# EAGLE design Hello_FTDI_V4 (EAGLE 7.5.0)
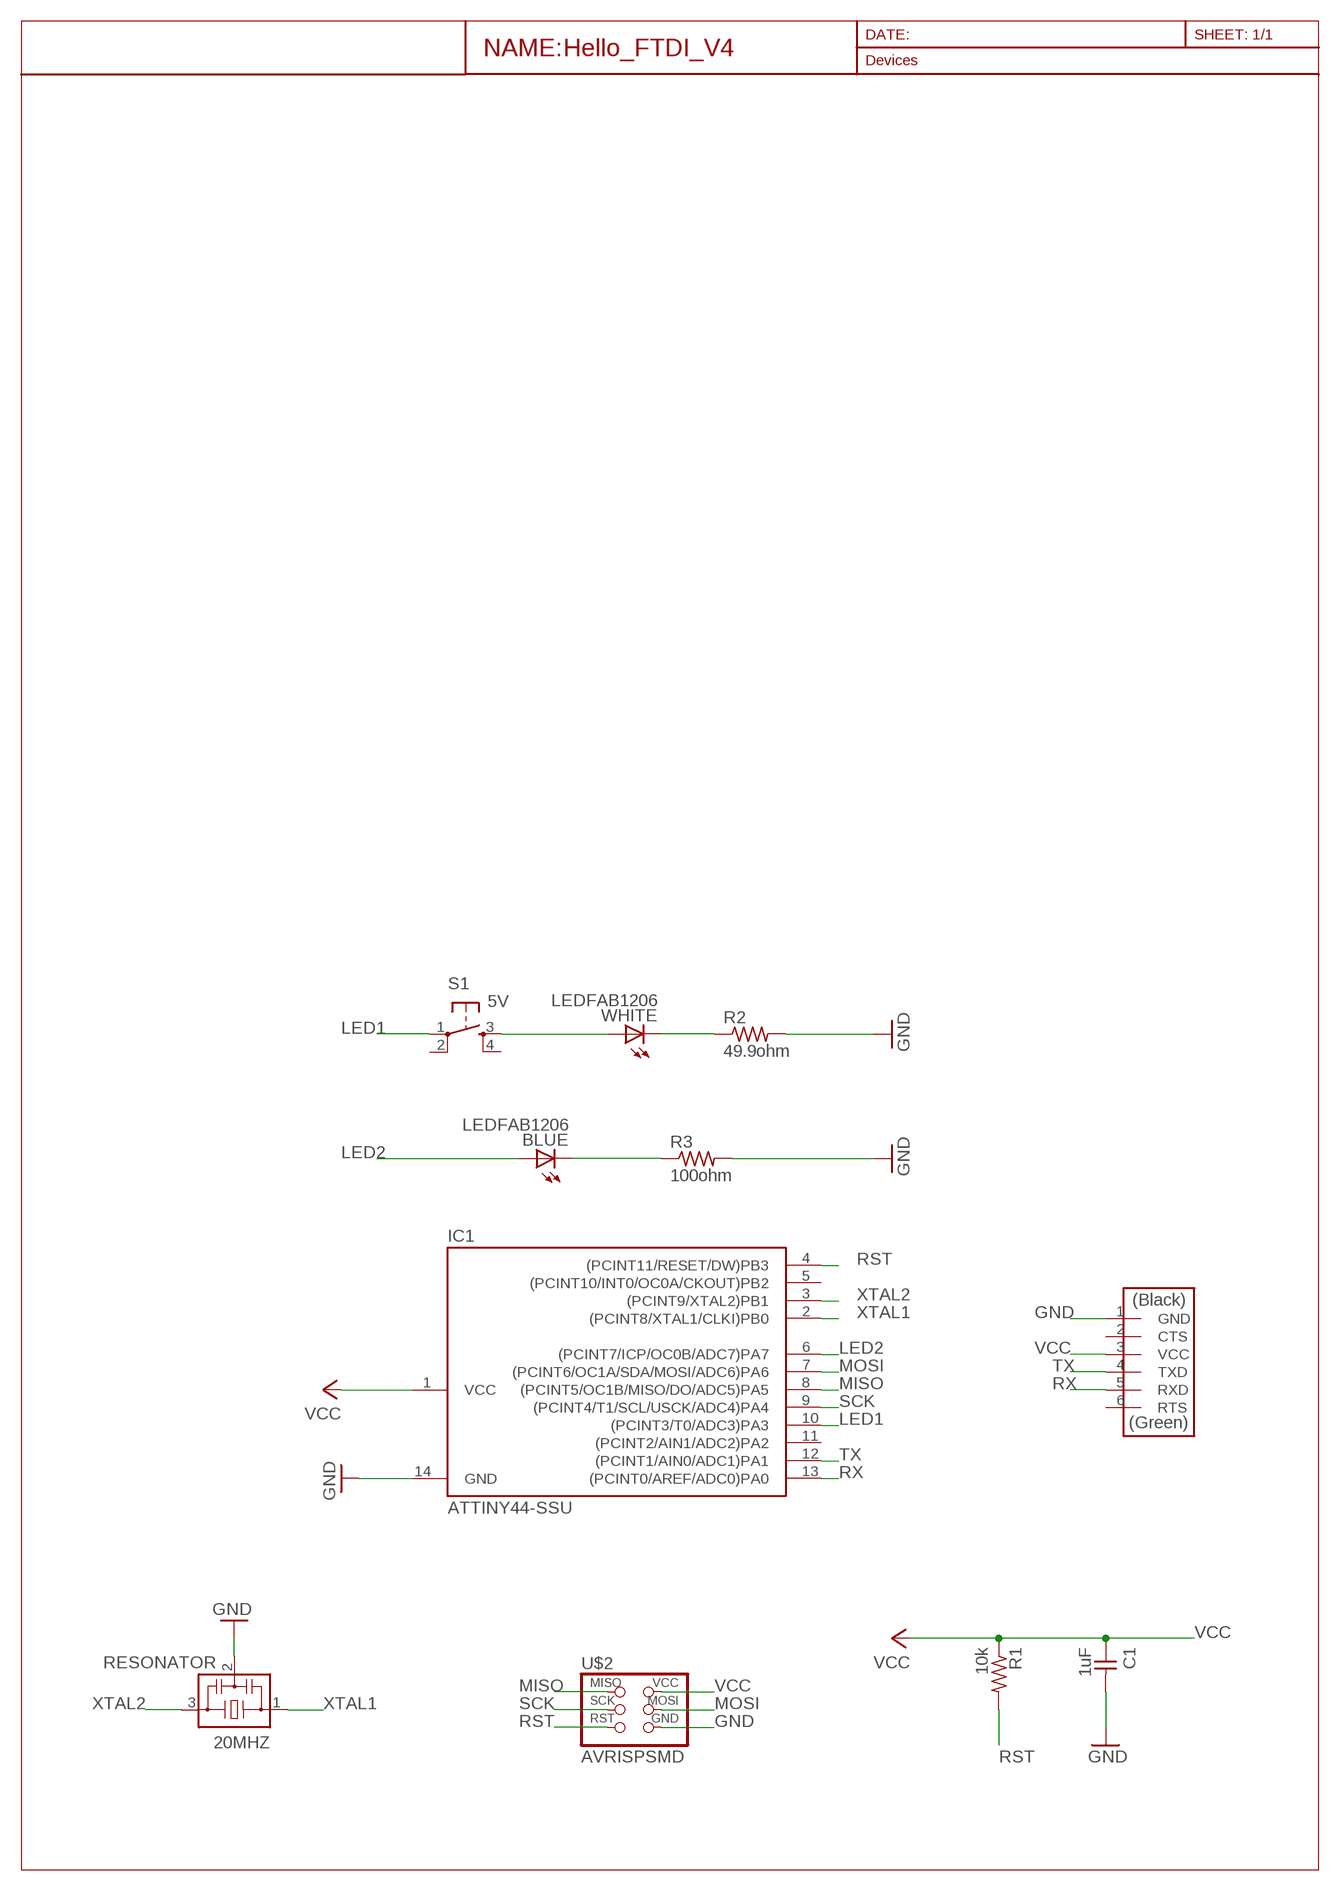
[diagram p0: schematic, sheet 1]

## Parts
20MHZ  RESONATOR  [EFOBM]
BLUE  LEDFAB1206  [LED1206FAB]
C1  1uF  CAP-UNPOLARIZEDFAB  [C1206FAB]
FTDI  FTDI-SMD-HEADER  [1X06SMD]
IC1  ATTINY44-SSU  [SOIC14]
R1  10k  RES-US1206FAB  [R1206FAB]
R2  49.9ohm  RES-US1206FAB  [R1206FAB]
R3  100ohm  RES-US1206FAB  [R1206FAB]
S1  5V  6MM_SWITCH6MM_SWITCH  [6MM_SWITCH]
U$2  AVRISPSMD  [2X03SMD]
WHITE  LEDFAB1206  [LED1206FAB]

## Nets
GND: 20MHZ.2 C1.2 FTDI.1(GND) IC1.14(GND) R2.2 R3.2 U$2.6(GND)
LED1: IC1.10((PCINT3/T0/ADC3)PA3) S1.1(P)
LED2: BLUE.1(A) IC1.6((PCINT7/ICP/OC0B/ADC7)PA7)
MISO: IC1.8((PCINT5/OC1B/MISO/DO/ADC5)PA5) U$2.1(MISO)
MOSI: IC1.7((PCINT6/OC1A/SDA/MOSI/ADC6)PA6) U$2.4(MOSI)
N$1: R2.1 WHITE.2(C)
N$2: S1.3(S) WHITE.1(A)
N$3: BLUE.2(C) R3.1
RST: IC1.4((PCINT11/RESET/DW)PB3) R1.2 U$2.5(RST)
RX: FTDI.5(RXD) IC1.13((PCINT0/AREF/ADC0)PA0)
SCK: IC1.9((PCINT4/T1/SCL/USCK/ADC4)PA4) U$2.3(SCK)
TX: FTDI.4(TXD) IC1.12((PCINT1/AIN0/ADC1)PA1)
VCC: C1.1 FTDI.3(VCC) IC1.1(VCC) R1.1 U$2.2(VCC)
XTAL1: 20MHZ.1 IC1.2((PCINT8/XTAL1/CLKI)PB0)
XTAL2: 20MHZ.3 IC1.3((PCINT9/XTAL2)PB1)
Unconnected: FTDI.2(CTS) FTDI.6(RTS) IC1.5((PCINT10/INT0/OC0A/CKOUT)PB2) IC1.11((PCINT2/AIN1/ADC2)PA2) S1.2(P1) S1.4(S1)

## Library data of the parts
20MHZ = fab:RESONATOR
BLUE WHITE = fab:LED: LED
C1 = fab:CAP-UNPOLARIZED
FTDI = fab:FTDI-SMD-HEADER
IC1 = fab:ATTINY44
R1-R3 = fab:RES-US: Resistor (US Symbol)
S1 = fab:6MM_SWITCH: OMRON SWITCH
U$2 = fab:AVRISP

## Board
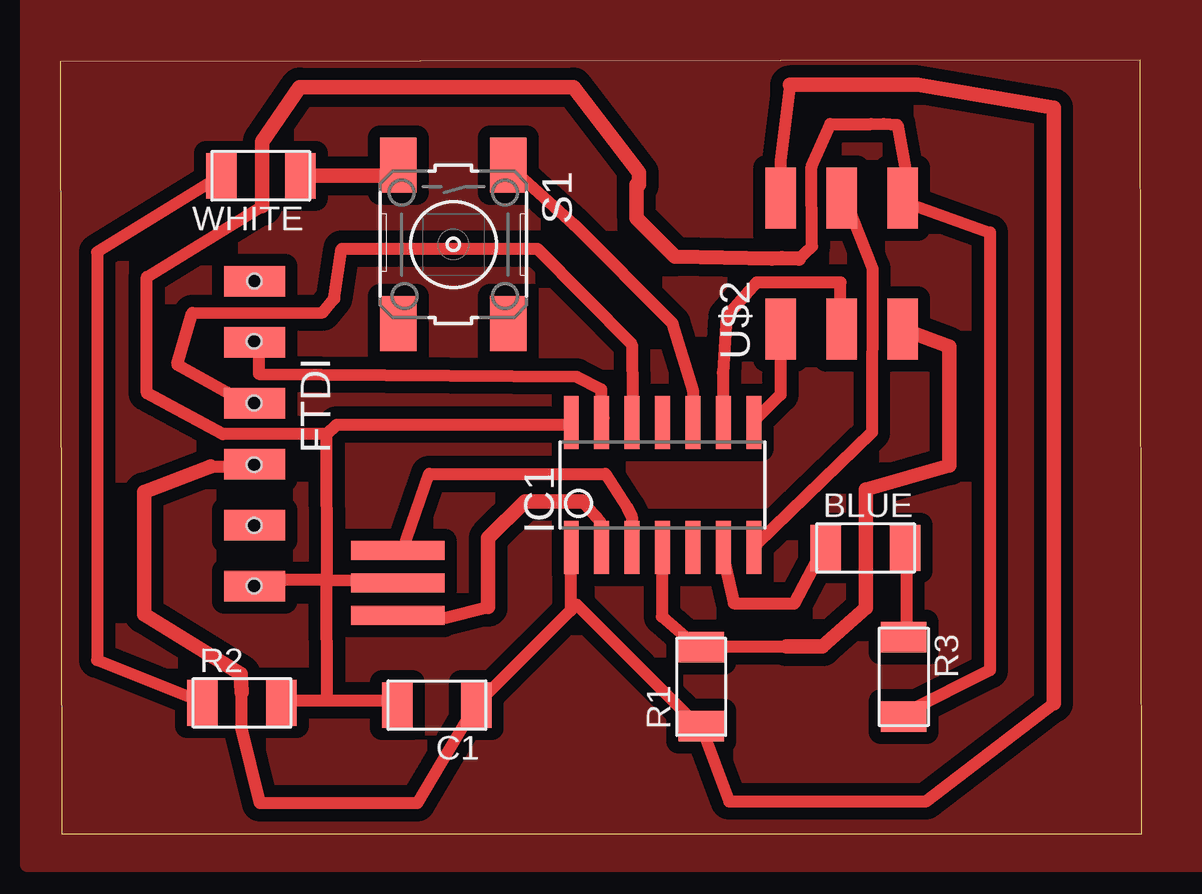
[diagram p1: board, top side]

Size 45.1 x 32.25 mm. Coordinates in mm from the lower left corner, seen from the top.
Outline: 0.06,0 45.1,0 45.04,32.25 0,32.19 0.06,0
Copper layers (1*16): Top 0.035mm / dielectric 1.5mm / Bottom 0.035mm
Design rules "default *": minimum track width 12mil, minimum drill 24mil, track to track 20mil, track to pad 16mil, pad to pad 16mil, via to via 16mil, smd to smd 8mil, copper to edge 0mil, drill to drill 40mil, minimum pad ring 10mil, minimum via ring 8mil, stop-mask expansion 4mil, vias tented up to drill 0mil, thermal gap 10mil
Holes 0.6 mm at 8.11,23.03 8.09,20.52 8.09,17.95 8.09,15.38 8.09,12.85 8.09,10.32

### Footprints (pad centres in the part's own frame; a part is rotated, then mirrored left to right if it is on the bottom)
EFOBM = smd 0.8 x 3.9: 1 -1.35,0; 2 0,0; 3 1.35,0
LED1206FAB = smd 1.27 x 1.905: 1 -1.651,0; 2 1.651,0
C1206FAB = smd 1.27 x 1.905: 1 -1.651,0; 2 1.651,0
1X06SMD = smd 2.54 x 1.27: 1 0,6.35; 2 0,3.81; 3 0,1.27; 4 0,-1.27; 5 0,-3.81; 6 0,-6.35
SOIC14 = smd 0.61 x 2.21: 1 -3.81,-2.603; 2 -2.54,-2.603; 3 -1.27,-2.603; 4 0,-2.603; 5 1.27,-2.603; 6 2.54,-2.603; 7 3.81,-2.603; 8 3.81,2.603; 9 2.54,2.603; 10 1.27,2.603; 11 0,2.603; 12 -1.27,2.603; 13 -2.54,2.603; 14 -3.81,2.603
R1206FAB = smd 1.27 x 1.905: 1 -1.651,0; 2 1.651,0
6MM_SWITCH = smd 2.286 x 1.524: 1 -3.302,2.286; 2 3.302,2.286; 3 -3.302,-2.286; 4 3.302,-2.286
2X03SMD = smd 2.54 x 1.27: 1 -2.54,2.54; 2 2.92,2.54; 3 -2.54,0; 4 2.92,0; 5 -2.54,-2.54; 6 2.92,-2.54

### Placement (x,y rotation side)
20MHZ  14.08,10.45 90 top
BLUE  33.58,11.91 0 top
C1  15.71,5.36 180 top
FTDI  8.11,16.67 180 top
IC1  25.12,14.54 0 top
R1  26.73,6.13 90 top
R2  7.59,5.45 0 top
R3  35.17,6.54 270 top
S1  16.4,24.56 270 top
U$2  32.58,23.57 90 top
WHITE  8.37,27.43 180 top

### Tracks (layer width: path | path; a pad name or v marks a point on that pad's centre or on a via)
GND
  Top 0.508: R3.2 35.29,5.05 38.77,6.81 38.77,25.06 35.29,26.3 U$2.6 35.29,27.48 34.9,29.55 34.33,29.59 33.81,29.59 32.11,29.59 31.33,27.8 31.35,24.48 30.8,23.98 | 11.14,5.55 9.29,5.55 R2.2 | 11.14,5.55 14.04,5.55 C1.2 | 11.14,5.55 11.11,10.57 | 11.11,10.57 11.13,10.57 | 11.13,10.57 11.12,16.65 | 11.12,16.65 11.54,17.05 21.29,17.05 IC1.14 | 11.11,10.57 8.23,10.57 FTDI.1 | 11.13,10.57 14.04,10.55 20MHZ.2 | 8.44,26.15 3.62,23.21 3.62,18.36 6.79,16.65 11.12,16.65
  Top 0.61: 30.8,23.98 30.09,24 29.68,23.98 25.64,24.05 24.04,25.65 24.04,27.05 24.14,27.05 24.14,27.55 21.4,31.12 10,31.12 8.44,28.85 8.44,26.15
LED1
  Top 0.508: S1.1 21.42,25.38 25.54,21.26 26.38,18.49 26.39,17.3 IC1.10
LED2
  Top 0.508: BLUE.1 31.79,11.8 30.61,9.59 28.09,9.6 27.69,11.4 IC1.6
MISO
  Top 0.508: IC1.8 29.04,17.3 30.04,18.3 30.04,20.8 U$2.1
MOSI
  Top 0.508: IC1.7 29.04,12.05 33.85,16.73 33.87,23.55 32.79,26.3 U$2.4
N$1
  Top 0.508: R2.1 5.79,5.55 1.55,7.23 1.55,24.23 6.54,27.3 WHITE.2
N$2
  Top 0.61: WHITE.1 13.67,27.43 S1.3
N$3
  Top 0.508: R3.1 35.29,8.3 35.29,11.8 BLUE.2
N$4
  pour Top: 48.29,-1.3 -1.36,-1.3 -1.36,34.77 48.01,34.77 48.01,-1.11
RST
  Top 0.508: IC1.4 25.09,11.8 25.09,9.05 26.54,7.8 R1.2 26.79,7.8 30.29,7.8 | 35.04,20.8 U$2.5
  Top 0.61: 30.29,7.8 31.79,7.8 33.59,9.41 33.59,14.34 37.08,15.35 37.08,20.3 U$2.5
RX
  Top 0.508: IC1.13 22.65,17.27 22.56,18.25 22.55,18.53 21.54,19.05 8.29,19.17 8.29,20.3 FTDI.5
SCK
  Top 0.508: IC1.9 27.63,19.21 27.79,21.55 29.04,22.97 32.54,22.97 32.54,21.05 U$2.3
TX
  Top 0.508: IC1.12 23.89,17.3 23.85,18.13 23.84,20.38 19.89,24.39 11.74,24.39 11.44,22.3 10.95,21.73 5.51,21.71 4.89,19.55 8.04,17.8 FTDI.4
VCC
  Top 0.508: 21.29,9.55 21.29,11.8 IC1.1 | 21.29,9.55 21.29,9.3 17.54,5.55 C1.1 17.29,5.3 14.89,1.27 8.34,1.27 7.57,4.39 7.57,5.89 | 21.29,9.55 21.54,9.55 26.54,4.55 R1.1 26.79,4.3 27.89,1.34 36.09,1.34 41.43,5.43 | 6.29,15.3 8.04,15.3 FTDI.3 | 30.42,31.22 30.04,28.05 30.04,26.55 U$2.2
  Top 0.61: 7.57,5.89 7.54,6.65 3.5,9.15 3.5,14.25 6.29,15.3 | 41.43,5.43 41.43,30.26 35.76,31.22 30.42,31.22
XTAL1
  Top 0.508: 21.79,13.85 22.35,13.21 22.53,12.99 22.54,12.05 IC1.2 | 17.85,9.44 16.04,9 14.29,9.1 20MHZ.1
  Top 0.61: 21.79,13.85 19.38,13.85 17.85,12.32 17.85,9.52 17.85,9.44
XTAL2
  Top 0.508: IC1.3 23.85,12.11 23.84,13.2 23.64,13.6 22.74,15 15.39,15 14.29,11.8 20MHZ.3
